FUNCTION_BLOCK FB_DO_IED_LD1_ATCC1_CtlV EXTENDS FB_AcsiCommonDataClass
VAR_INPUT
	mag: FB_AcsiDATypeAnalogueValue := (fc:=ACSI_FC_MX, TrgOp:=ACSI_TrgOp_dchg OR ACSI_TrgOp_dupd, bLinkResult:=THIS^.AddDataToContainer(ipData:=mag));
	q: FB_AcsiDATypeQuality := (fc:=ACSI_FC_MX, TrgOp:=ACSI_TrgOp_qchg, bLinkResult:=THIS^.AddDataToContainer(ipData:=q));
	t: FB_AcsiDATypeTimeStamp := (fc:=ACSI_FC_MX, bLinkResult:=THIS^.AddDataToContainer(ipData:=t));
END_VAR
VAR
END_VAR

END_FUNCTION_BLOCK
